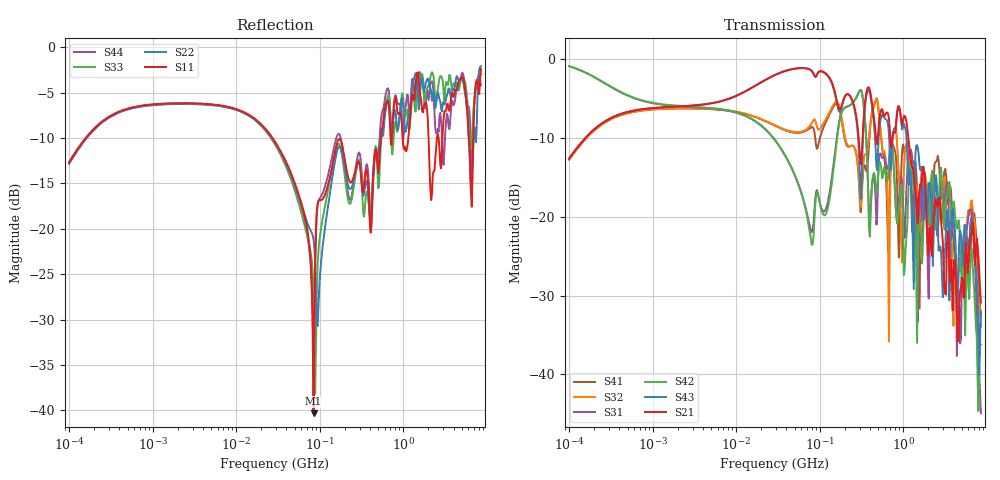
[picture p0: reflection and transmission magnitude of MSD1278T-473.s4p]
# MHz S MA R 50
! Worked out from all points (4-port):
!   498 points, 100 kHz to 8.5 GHz, reference 50 ohm
!   strongest paths, dB at 100 kHz, 1.698 MHz, 29.49 MHz, 500.7 MHz, 8.5 GHz:
!     S21: -12.6, -6.0, -2.0, -9.4, -30.9
!     S43: -12.6, -6.0, -2.0, -11.5, -32.0
!     S42: -0.9, -5.8, -10.3, -14.8, -36.2
!     S31: -0.9, -5.9, -10.4, -14.9, -44.9
!     S32: -12.7, -6.3, -8.4, -6.0, -31.9
!     S41: -12.8, -6.3, -8.5, -5.9, -33.9
!   lowest |S11| = -40.3 dB at 84.32 MHz (marker M1), VSWR 1.02, Z = 49.1 - j0.394 ohm
!   |S11| at or under -10 dB: 27.35 MHz to 539.4 MHz (512 MHz wide, 181 % of centre); 2.009 GHz to 2.531 GHz (522.2 MHz wide, 23 % of centre); 6.108 GHz to 6.897 GHz (788.4 MHz wide, 12.1 % of centre)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
0.1  0.2326 60.0  0.2342 60.9  0.903 -13.2  0.2303 -119.7
     0.2342 60.9  0.228 60.3  0.2308 -119.6  0.9043 -13.1
     0.903 -13.2  0.2308 -119.6  0.2322 60.4  0.2343 60.8
     0.2303 -119.7  0.9043 -13.1  0.2343 60.8  0.2302 60.5
15.20675  0.4166 -30.8  0.6567 13.4  0.4177 -36.6  0.4384 140.3
          0.6567 13.4  0.412 -32.9  0.4398 138.4  0.4203 -36.3
          0.4177 -36.6  0.4398 138.4  0.4125 -32.9  0.6578 13.3
          0.4384 140.3  0.4203 -36.3  0.6578 13.3  0.411 -31.0
84.31651  0.009637 -155.4  0.8081 -25.8  0.09193 -74.9  0.3643 50.5
          0.8081 -25.8  0.08738 -96.4  0.4114 56.4  0.07587 -62.3
          0.09193 -74.9  0.4114 56.4  0.04754 -86.7  0.8119 -26.9
          0.3643 50.5  0.07587 -62.3  0.8119 -26.9  0.01535 -143.8
302.9285  0.223 50.3  0.2439 -66.7  0.6359 -39.5  0.1244 -46.0
          0.2439 -66.7  0.2265 49.6  0.1334 -41.8  0.6352 -40.8
          0.6359 -39.5  0.1334 -41.8  0.2348 30.9  0.1773 -81.2
          0.1244 -46.0  0.6352 -40.8  0.1773 -81.2  0.2575 31.9
5026.862  0.685 -96.2  0.04125 -128.7  0.03783 -70.2  0.05425 -134.8
          0.04125 -128.7  0.6604 -101.0  0.04821 -84.5  0.03636 176.2
          0.03783 -70.2  0.04821 -84.5  0.6829 -101.5  0.06755 -166.0
          0.05425 -134.8  0.03636 176.2  0.06755 -166.0  0.72 -89.6
6462.473  0.1589 154.1  0.07843 54.6  0.112 48.8  0.06752 133.6
          0.07843 54.6  0.1625 148.0  0.1247 104.2  0.06003 50.8
          0.112 48.8  0.1247 104.2  0.2747 99.5  0.09743 36.4
          0.06752 133.6  0.06003 50.8  0.09743 36.4  0.282 -153.5
8500  0.7609 -43.6  0.02863 -126.8  0.005672 -27.8  0.02025 -152.5
      0.02863 -126.8  0.7868 -43.8  0.02547 -115.2  0.01551 -47.4
      0.005672 -27.8  0.02547 -115.2  0.7108 -53.0  0.02499 -24.7
      0.02025 -152.5  0.01551 -47.4  0.02499 -24.7  0.6188 -47.2
